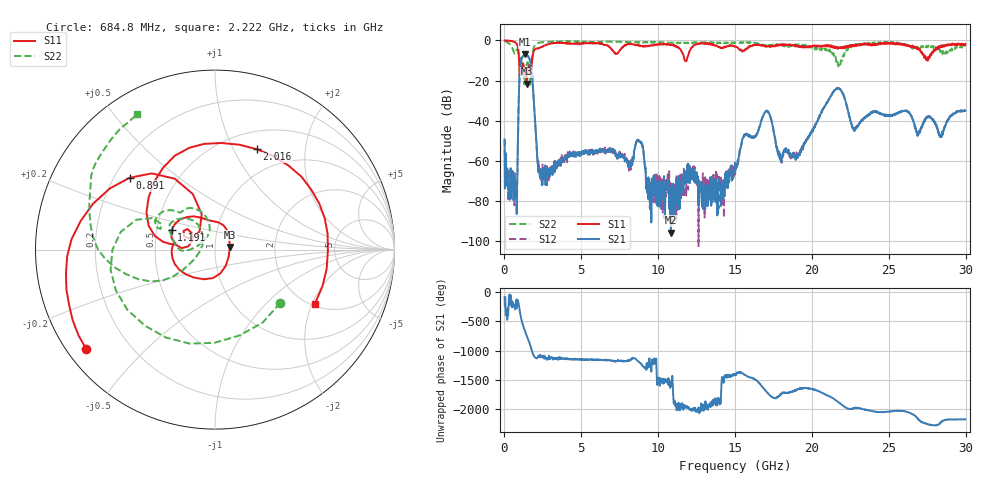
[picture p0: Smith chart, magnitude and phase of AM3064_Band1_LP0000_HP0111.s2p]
# Hz S DB R 50.0
!freq dBS11 angS11 dBS21 angS21 dBS12 angS12 dBS22 angS22
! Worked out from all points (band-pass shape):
!   1600 points, 10 MHz to 29.98 GHz, reference 50 ohm
!   highest |S21| = -6.93 dB at 1.36 GHz (marker M1); lowest = -95.9 dB at 10.83 GHz (marker M2)
!   |S21| within 3 dB of the highest: 1.089 GHz to 1.661 GHz (572.1 MHz wide, 41.6 % of centre)
!   lowest |S11| = -21.6 dB at 1.435 GHz (marker M3), VSWR 1.18, Z = 58.9 + j1.78 ohm
!   |S11| at or under -10 dB: 949.3 MHz to 1.8 GHz (850.5 MHz wide, 61.9 % of centre); 11.74 GHz to 11.85 GHz (104 MHz wide, 0.882 % of centre); 27.52374 GHz to 27.5387 GHz (14.96 MHz wide, 0.0543 % of centre)
!   |S22| runs from -22.6 to -0.2 dB; largest |S21 - S12| = 0.0064
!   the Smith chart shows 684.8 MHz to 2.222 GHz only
!   S11 on the Smith chart (normalised r, x): 684.8 MHz: 0.05, -0.34; 891 MHz: 0.26, +0.34; 1.191 GHz: 0.60, +0.14; 2.016 GHz: 0.70, +1.24; 2.222 GHz: 2.07, -2.10
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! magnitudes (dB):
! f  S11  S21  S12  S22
! 10 MHz  0.0  -49.5  -49.2  -0.2
! 684.8 MHz  -0.9  -73.4  -69.2  -6.6
! 891 MHz  -4.1  -43.6  -43.6  -5.4
! 1.191 GHz  -11.5  -8.0  -7.9  -11.9
! 1.36 GHz  -16.4  -6.9  -6.9  -15.7
! 1.435 GHz  -21.6  -7.1  -7.1  -12.5
! 1.734 GHz  -13.4  -12.6  -12.5  -15.5
! 2.016 GHz  -4.4  -43.7  -43.2  -2.1
! 2.222 GHz  -4.0  -61.9  -64.6  -1.2
! 5.015 GHz  -1.4  -56.1  -57.2  -0.8
! 8.763 GHz  -2.8  -50.3  -49.9  -1.1
! 9.363 GHz  -2.8  -68.3  -80.2  -1.0
! 10 GHz  -2.0  -82.8  -71.0  -0.9
! 10.83 GHz  -2.0  -95.9  -77.7  -1.0
! 15 GHz  -3.0  -61.0  -66.9  -1.2
! 17.01 GHz  -3.2  -35.3  -35.3  -2.4
! 17.93 GHz  -2.0  -56.5  -58.0  -1.9
! 19.99 GHz  -3.2  -45.4  -45.5  -3.4
! 21.66 GHz  -3.9  -23.8  -23.8  -9.9
! 22.73 GHz  -2.7  -45.0  -44.2  -2.2
! 25 GHz  -1.2  -37.6  -37.5  -1.1
! 29.98 GHz  -1.8  -35.1  -35.1  -3.1
